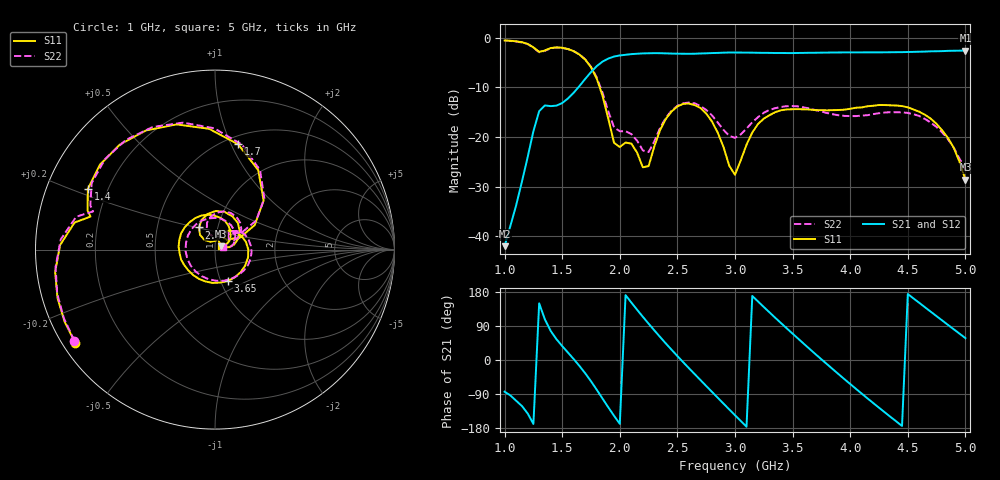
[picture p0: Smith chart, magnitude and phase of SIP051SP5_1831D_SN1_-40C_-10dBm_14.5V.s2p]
# GHz  S  dB  R  50
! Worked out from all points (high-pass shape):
!   81 points, 1 GHz to 5 GHz, reference 50 ohm
!   highest |S21| = -2.61 dB at 5 GHz (marker M1); lowest = -42.0 dB at 1 GHz (marker M2)
!   |S21| within 3 dB of the highest: 1.807 GHz to end of sweep
!   lowest |S11| = -28.6 dB at 5 GHz (marker M3), VSWR 1.08, Z = 53.2 + j2.13 ohm
!   |S11| at or under -10 dB: 1.825 GHz to end of sweep
!   |S22| runs from -26.6 to -0.6 dB; largest |S21 - S12| = 0.002
!   S11 on the Smith chart (normalised r, x): 1 GHz: 0.04, -0.30; 1.4 GHz: 0.13, +0.22; 1.7 GHz: 0.58, +1.06; 2.4 GHz: 0.81, +0.21; 3.65 GHz: 1.08, -0.39; 5 GHz: 1.06, +0.04
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1  -0.57 -146.2  -41.98 -83.7  -41.87 -84.4  -0.59 -147.1
1.3  -2.88 165.2  -14.82 149.5  -14.79 149.7  -2.96 162.6
1.4  -2.10 154.5  -13.79 76.7  -13.81 77.0  -2.15 151.6
1.7  -4.42 77.6  -8.31 -35.1  -8.32 -35.2  -4.39 75.5
1.85  -11.71 31.6  -4.83 -101.8  -4.83 -101.8  -11.07 35.1
1.95  -21.19 40.4  -3.81 -147.2  -3.83 -147.1  -18.05 44.2
2.05  -21.13 77.2  -3.46 171.2  -3.46 171.2  -18.83 63.3
2.25  -25.86 120.7  -3.15 95.9  -3.15 95.9  -23.05 93.5
2.35  -18.60 135.5  -3.14 60.6  -3.14 60.6  -18.16 111.6
2.4  -16.36 125.8  -3.18 43.5  -3.17 43.5  -16.12 106.6
2.55  -13.34 88.8  -3.25 -5.7  -3.25 -5.7  -13.23 77.4
2.75  -15.28 37.1  -3.17 -68.6  -3.16 -68.5  -14.56 38.5
3  -27.61 48.5  -3.01 -145.8  -2.99 -145.8  -20.17 40.0
3.15  -19.11 63.2  -3.03 169.1  -3.04 169.0  -17.04 46.6
3.35  -15.01 13.7  -3.10 111.3  -3.10 111.3  -14.20 16.6
3.65  -14.48 -67.8  -3.06 28.6  -3.06 28.6  -14.30 -47.8
3.7  -14.60 -81.2  -3.05 15.1  -3.04 15.2  -14.60 -60.7
4.05  -14.12 -163.6  -2.98 -76.1  -2.98 -76.1  -15.80 -162.0
4.35  -13.63 133.0  -2.95 -150.2  -2.95 -150.2  -15.02 113.8
4.55  -14.47 90.9  -2.87 162.3  -2.87 162.4  -15.43 66.8
4.75  -17.39 51.2  -2.75 115.6  -2.75 115.6  -18.02 26.9
5  -28.61 32.7  -2.61 57.7  -2.62 57.6  -26.61 16.2
